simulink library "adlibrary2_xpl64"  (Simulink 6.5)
undefined symbols (not defined in the file or in its folder): Bit, Black, blackbox2, blue, Box, clock_ratio, ddcd732b, gcbh, Inactive, lbif64_xpl_config, Location, Lower, program, VER_STRING_GOES_HERE, white, Width, xbsIndex_r4, xlBlockLoadCallback
libraries: xbsIndex_r4 x49, adlibrary2_xpl64 x1

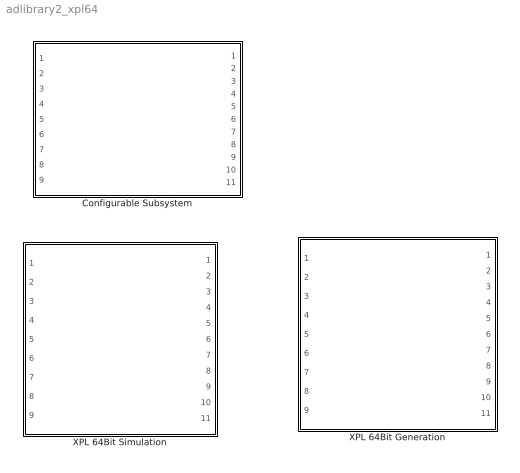
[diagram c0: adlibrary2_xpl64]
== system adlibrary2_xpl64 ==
  Configurable Subsystem : Subsystem  Tag=configX  BlockChoice=XPL 64Bit Simulation  mask{program=program, clock_ratio=clock_ratio}
      mask prompts: program "Local Bus Script Program"; clock_ratio "Clock Ratio"
  XPL 64Bit Generation : Subsystem
  XPL 64Bit Simulation : Subsystem  mask{program=program, clock_ratio=clock_ratio}
      mask prompts: program "Local Bus Script Program"; clock_ratio "Clock Ratio"

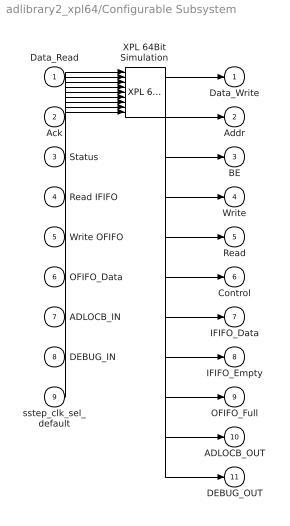
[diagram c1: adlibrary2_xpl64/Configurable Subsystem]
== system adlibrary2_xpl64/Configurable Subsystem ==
  Data_Read : Inport
  Ack : Inport  Port=2
  Status : Inport  Port=3
  Read IFIFO : Inport  Port=4
  Write OFIFO : Inport  Port=5
  OFIFO_Data : Inport  Port=6
  ADLOCB_IN : Inport  Port=7
  DEBUG_IN : Inport  Port=8
  sstep_clk_sel_default : Inport  Port=9
  XPL 64Bit Simulation : adlibrary2_xpl64/XPL 64Bit Simulation  SystemSampleTime=-1  program=program  clock_ratio=clock_ratio
  Data_Write : Outport
  Addr : Outport  Port=2
  BE : Outport  Port=3
  Write : Outport  Port=4
  Read : Outport  Port=5
  Control : Outport  Port=6
  IFIFO_Data : Outport  Port=7
  IFIFO_Empty : Outport  Port=8
  OFIFO_Full : Outport  Port=9
  ADLOCB_OUT : Outport  Port=10
  DEBUG_OUT : Outport  Port=11
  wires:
  Data_Read/1 -> XPL 64Bit Simulation/1
  Ack/1 -> XPL 64Bit Simulation/2
  Status/1 -> XPL 64Bit Simulation/3
  Read IFIFO/1 -> XPL 64Bit Simulation/4
  Write OFIFO/1 -> XPL 64Bit Simulation/5
  OFIFO_Data/1 -> XPL 64Bit Simulation/6
  ADLOCB_IN/1 -> XPL 64Bit Simulation/7
  DEBUG_IN/1 -> XPL 64Bit Simulation/8
  sstep_clk_sel_default/1 -> XPL 64Bit Simulation/9
  XPL 64Bit Simulation/1 -> Data_Write/1
  XPL 64Bit Simulation/2 -> Addr/1
  XPL 64Bit Simulation/3 -> BE/1
  XPL 64Bit Simulation/4 -> Write/1
  XPL 64Bit Simulation/5 -> Read/1
  XPL 64Bit Simulation/6 -> Control/1
  XPL 64Bit Simulation/7 -> IFIFO_Data/1
  XPL 64Bit Simulation/8 -> IFIFO_Empty/1
  XPL 64Bit Simulation/9 -> OFIFO_Full/1
  XPL 64Bit Simulation/10 -> ADLOCB_OUT/1
  XPL 64Bit Simulation/11 -> DEBUG_OUT/1

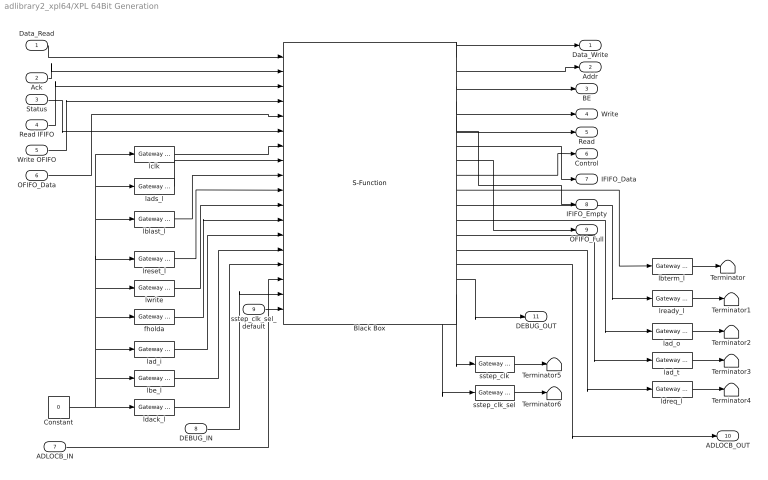
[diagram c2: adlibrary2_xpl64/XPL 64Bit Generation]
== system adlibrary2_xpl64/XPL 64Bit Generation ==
  Data_Read : Inport
  Ack : Inport  Port=2
  Status : Inport  Port=3
  Read IFIFO : Inport  Port=4
  Write OFIFO : Inport  Port=5
  OFIFO_Data : Inport  Port=6
  ADLOCB_IN : Inport  Port=7
  DEBUG_IN : Inport  Port=8
  sstep_clk_sel_default : Inport  Port=9
  Black Box : S-Function  AncestorBlock=xbsIndex_r4/Black Box  LoadFcn=xlBlockLoadCallback(gcbh);  FunctionName=sysgen  Parameters=ptable_  mask(Xilinx Black Box Block){infoedit=Incorporates black box HDL and simulation model into a System Generator design.<P><P>You must supply a Black Box with certain information about the HDL component you would like to bring into System Generator. This information is provided through a Matlab function.<P><P>When "Simulation mode" is set to "Inactive", you will typically want to provide a separate simulation model by using a Simulation 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, init_code=lbif64_xpl_config, sim_method=Inactive, sim_method_sgadvanced=, engine_block=, xl_use_area=on, xl_use_area_sgadvanced=, xl_area=[576,805, 3, 586, 0, 0, 162], block_version=VER_STRING_GOES_HERE, has_advanced_control=0, sggui_pos=20,20,356,367, block_type=blackbox2, sg_icon_stat=240,390,18,18,white,blue,0,ddcd732b, sg_mask_display=fprintf('','COMMENT: begin icon graphics '); patch([0 240 240 0 ],[0 0 390 390 ],[0.77 0.82 0.91]); patch([56 16 72 16 56 119 136 153 221 167 116 79 135 79 116 167 221 153 136 119 56 ],[101 141 197 253 293 293 276 293 293 239 290 253 197 141 104 155 101 101 118 101 101 ],[0.98 0.96 0.92]); plot([0 0 240 240 0 ],[0 390 390 0 0 ]); fprintf('','COMMENT: end icon graphics');  fprintf('','COMMENT: begi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, sg_list_contents=}
      mask prompts: infoedit ""; init_code "Block configuration m-function"; sim_method "Simulation mode"; engine_block "HDL co-simulator to use  (specify helper block by name)"; xl_use_area "Define FPGA area for resource estimation"; xl_area "FPGA area [slices, FFs, BRAMs, LUTs, IOBs, emb. mults, TBUFs]"; block_version ""; has_advanced_control ""; sggui_pos ""; block_type ""; sg_icon_stat ""; sg_mask_display ""; sg_list_contents ""
      mask help: Incorporates black box HDL and simulation model into a System Generator design. You must supply a Black Box with certain information about the HDL component you would like to bring into System Generator. This information is provided through a Matlab function. When "Simulation mode" is set to "Inactive", you will typically want to provide a separate simulation model by using a Simulation Multiplexer. When "Simulation mode" is set to "External co-simulator", you must include a ModelSim block in the design.
      mask init:
      | xlMungeMaskParams;
      | 
      | mdlPath = xlGetMdlDir(bdroot);
      | 
      | refBlk = get_param(gcb,'referenceBlock');
      | if (isempty(refBlk) | strncmp(refBlk,'xbsIndex',8))
      | srcPath = mdlPath;
      | else
      | srcPath = xlPathToReference;
      | if (isempty(srcPath))
      | srcPath = mdlPath;
      | end
      | end
      | 
      | if (sim_method==3)
      | validEngineBlock = 0;
      | try
      | engineBlock = xlBlockNameRelPath(get_param(gcb,'Parent'),engine_block);
      | catch
      | engineBlock = '//';
      | end
      | try 
      | engineWorkDir = get_param(engineBlock,'dir');
      | validEngineBlock = 1;
      | engine_handle = get_param(engineBlock,'Handle');
      | catch
      | end
      | end
      | 
      | % build black box config function
      | block_config = ['sysgen:black_box_config:' init_code];
      | 
      | serialized_declarations = '{''engine_handle''=>''Double'',''sim_method''=>''Int'',''validEngineBlock''=>''Int'',''engineWorkDir''=>''String'',''engine_block''=>''String'',''init_code''=>''String'',''mdlPath''=>''String'',''srcPath''=>''String'',''block_config''=>''String'',}';
      | ptable_ = xlblockprep(get_param(gcb, 'MaskWSVariables'));
  Constant : Constant  Value=0  OutDataType=sfix(16)  ConRadixGroup=Use specified scaling  OutScaling=2^0  SampleTime=inf  FramePeriod=inf
  Terminator{,1..6} (7 alike) : Terminator
  fholda : xbsIndex_r4/Gateway In  arith_type=Boolean  n_bits=8  bin_pt=6  quantization="Round  (unbiased: +/- Inf)"  overflow=Saturate  period=1  dbl_ovrd=off  timing_constraint=None  locs_specified=off  LOCs={}  block_type=gatewayin
  lad_i : xbsIndex_r4/Gateway In  arith_type=Unsigned  n_bits=64  bin_pt=0  quantization="Round  (unbiased: +/- Inf)"  overflow=Saturate  period=1  dbl_ovrd=off  timing_constraint=None  locs_specified=off  LOCs={}  block_type=gatewayin
  lad_o : xbsIndex_r4/Gateway Out  hdl_port=on  timing_constraint=None  locs_specified=off  LOCs={}  block_type=gatewayout
  lad_t : xbsIndex_r4/Gateway Out  hdl_port=on  timing_constraint=None  locs_specified=off  LOCs={}  block_type=gatewayout
  lads_l : xbsIndex_r4/Gateway In  arith_type=Boolean  n_bits=8  bin_pt=6  quantization="Round  (unbiased: +/- Inf)"  overflow=Saturate  period=1  dbl_ovrd=off  timing_constraint=None  locs_specified=off  LOCs={}  block_type=gatewayin
  lbe_l : xbsIndex_r4/Gateway In  arith_type=Unsigned  n_bits=8  bin_pt=0  quantization="Round  (unbiased: +/- Inf)"  overflow=Saturate  period=1  dbl_ovrd=off  timing_constraint=None  locs_specified=off  LOCs={}  block_type=gatewayin
  lblast_l : xbsIndex_r4/Gateway In  arith_type=Boolean  n_bits=8  bin_pt=6  quantization="Round  (unbiased: +/- Inf)"  overflow=Saturate  period=1  dbl_ovrd=off  timing_constraint=None  locs_specified=off  LOCs={}  block_type=gatewayin
  lbterm_l : xbsIndex_r4/Gateway Out  hdl_port=on  timing_constraint=None  locs_specified=off  LOCs={}  block_type=gatewayout
  lclk : xbsIndex_r4/Gateway In  arith_type=Boolean  n_bits=8  bin_pt=6  quantization="Round  (unbiased: +/- Inf)"  overflow=Saturate  period=1  dbl_ovrd=off  timing_constraint=None  locs_specified=off  LOCs={}  block_type=gatewayin
  ldack_l : xbsIndex_r4/Gateway In  arith_type=Unsigned  n_bits=2  bin_pt=0  quantization="Round  (unbiased: +/- Inf)"  overflow=Saturate  period=1  dbl_ovrd=off  timing_constraint=None  locs_specified=off  LOCs={}  block_type=gatewayin
  ldreq_l : xbsIndex_r4/Gateway Out  hdl_port=on  timing_constraint=None  locs_specified=off  LOCs={}  block_type=gatewayout
  lready_l : xbsIndex_r4/Gateway Out  hdl_port=on  timing_constraint=None  locs_specified=off  LOCs={}  block_type=gatewayout
  lreset_l : xbsIndex_r4/Gateway In  arith_type=Boolean  n_bits=8  bin_pt=6  quantization="Round  (unbiased: +/- Inf)"  overflow=Saturate  period=1  dbl_ovrd=off  timing_constraint=None  locs_specified=off  LOCs={}  block_type=gatewayin
  lwrite : xbsIndex_r4/Gateway In  arith_type=Boolean  n_bits=8  bin_pt=6  quantization="Round  (unbiased: +/- Inf)"  overflow=Saturate  period=1  dbl_ovrd=off  timing_constraint=None  locs_specified=off  LOCs={}  block_type=gatewayin
  sstep_clk : xbsIndex_r4/Gateway Out  hdl_port=on  timing_constraint=None  locs_specified=off  LOCs={}  block_type=gatewayout
  sstep_clk_sel : xbsIndex_r4/Gateway Out  hdl_port=on  timing_constraint=None  locs_specified=off  LOCs={}  block_type=gatewayout
  Data_Write : Outport
  Addr : Outport  Port=2
  BE : Outport  Port=3
  Write : Outport  Port=4
  Read : Outport  Port=5
  Control : Outport  Port=6
  IFIFO_Data : Outport  Port=7
  IFIFO_Empty : Outport  Port=8
  OFIFO_Full : Outport  Port=9
  ADLOCB_OUT : Outport  Port=10
  DEBUG_OUT : Outport  Port=11
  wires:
  lbe_l/1 -> Black Box/14
  Data_Read/1 -> Black Box/1
  Ack/1 -> Black Box/2
  Status/1 -> Black Box/6
  Read IFIFO/1 -> Black Box/3
  Write OFIFO/1 -> Black Box/4
  OFIFO_Data/1 -> Black Box/5
  Black Box/1 -> Data_Write/1
  Black Box/2 -> Addr/1
  lclk/1 -> Black Box/7
  lads_l/1 -> Black Box/8
  lblast_l/1 -> Black Box/9
  lreset_l/1 -> Black Box/10
  lwrite/1 -> Black Box/11
  fholda/1 -> Black Box/12
  lad_i/1 -> Black Box/13
  ldack_l/1 -> Black Box/15
  Constant/1 -> ldack_l/1, lclk/1, lads_l/1, lblast_l/1, lreset_l/1, lwrite/1, fholda/1, lad_i/1, lbe_l/1
  lbterm_l/1 -> Terminator/1
  lready_l/1 -> Terminator1/1
  lad_o/1 -> Terminator2/1
  lad_t/1 -> Terminator3/1
  ldreq_l/1 -> Terminator4/1
  Black Box/14 -> ldreq_l/1
  Black Box/3 -> BE/1
  Black Box/4 -> Write/1
  Black Box/5 -> Read/1
  Black Box/6 -> IFIFO_Empty/1
  Black Box/7 -> IFIFO_Data/1
  Black Box/8 -> OFIFO_Full/1
  Black Box/9 -> Control/1
  Black Box/10 -> lbterm_l/1
  Black Box/11 -> lready_l/1
  Black Box/12 -> lad_o/1
  Black Box/13 -> lad_t/1
  Black Box/15 -> ADLOCB_OUT/1
  ADLOCB_IN/1 -> Black Box/16
  sstep_clk/1 -> Terminator5/1
  sstep_clk_sel/1 -> Terminator6/1
  DEBUG_IN/1 -> Black Box/17
  Black Box/17 -> sstep_clk/1
  Black Box/18 -> sstep_clk_sel/1
  Black Box/16 -> DEBUG_OUT/1
  sstep_clk_sel_default/1 -> Black Box/18

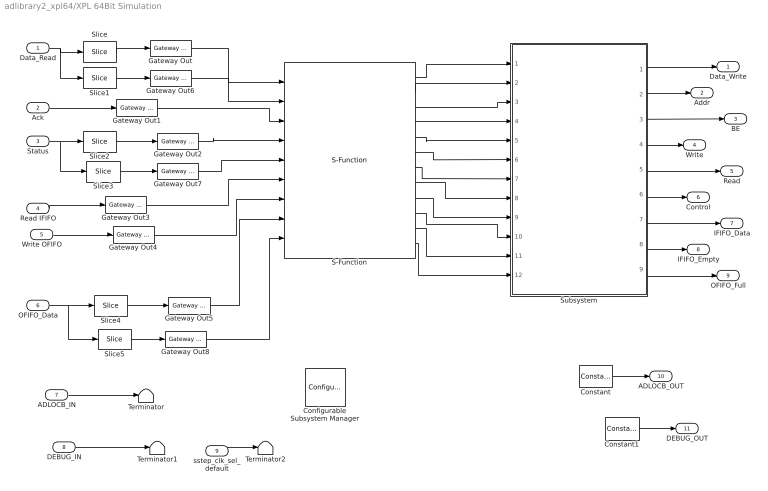
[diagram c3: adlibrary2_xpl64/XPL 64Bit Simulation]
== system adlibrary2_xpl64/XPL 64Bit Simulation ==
  Data_Read : Inport
  Ack : Inport  Port=2
  Status : Inport  Port=3
  Read IFIFO : Inport  Port=4
  Write OFIFO : Inport  Port=5
  OFIFO_Data : Inport  Port=6
  ADLOCB_IN : Inport  Port=7
  DEBUG_IN : Inport  Port=8
  sstep_clk_sel_default : Inport  Port=9
  Configurable Subsystem Manager : xbsIndex_r4/Configurable Subsystem Manager  Tag=xcfgMgr  block_type=configsubsys
  Constant : xbsIndex_r4/Constant  arith_type=Unsigned  const=0  n_bits=66  bin_pt=0  explicit_period=on  period=ad_get_simulink_period  equ=P=C  opselect=C  inp2=PCIN>>17  opr=+  inp1=P  carry=CIN  dbl_ovrd=off  block_type=constant
  Constant1 : xbsIndex_r4/Constant  arith_type=Unsigned  const=0  n_bits=40  bin_pt=0  explicit_period=on  period=ad_get_simulink_period  equ=P=C  opselect=C  inp2=PCIN>>17  opr=+  inp1=P  carry=CIN  dbl_ovrd=off  block_type=constant
  Gateway Out{,1..8} (9 alike) : xbsIndex_r4/Gateway Out  hdl_port=off  timing_constraint=None  locs_specified=off  LOCs={}  block_type=gatewayout
  S-Function : S-Function  FunctionName=lbif_xpl64  Parameters=program,clock_ratio
  Slice : xbsIndex_r4/Slice  nbits=32  boolean_output=off  mode=Lower Bit Location + Width  bit1=0  base1=MSB of Input  bit0=0  base0=LSB of Input  dbl_ovrd=off  block_type=slice
  Slice1 : xbsIndex_r4/Slice  nbits=32  boolean_output=off  mode=Lower Bit Location + Width  bit1=0  base1=MSB of Input  bit0=32  base0=LSB of Input  dbl_ovrd=off  block_type=slice
  Slice2 : xbsIndex_r4/Slice  nbits=32  boolean_output=off  mode=Lower Bit Location + Width  bit1=0  base1=MSB of Input  bit0=0  base0=LSB of Input  dbl_ovrd=off  block_type=slice
  Slice3 : xbsIndex_r4/Slice  nbits=32  boolean_output=off  mode=Lower Bit Location + Width  bit1=0  base1=MSB of Input  bit0=32  base0=LSB of Input  dbl_ovrd=off  block_type=slice
  Slice4 : xbsIndex_r4/Slice  nbits=32  boolean_output=off  mode=Lower Bit Location + Width  bit1=0  base1=MSB of Input  bit0=0  base0=LSB of Input  dbl_ovrd=off  block_type=slice
  Slice5 : xbsIndex_r4/Slice  nbits=32  boolean_output=off  mode=Lower Bit Location + Width  bit1=0  base1=MSB of Input  bit0=32  base0=LSB of Input  dbl_ovrd=off  block_type=slice
  Subsystem : Subsystem
  Terminator : Terminator
  Terminator1 : Terminator
  Terminator2 : Terminator
  Data_Write : Outport
  Addr : Outport  Port=2
  BE : Outport  Port=3
  Write : Outport  Port=4
  Read : Outport  Port=5
  Control : Outport  Port=6
  IFIFO_Data : Outport  Port=7
  IFIFO_Empty : Outport  Port=8
  OFIFO_Full : Outport  Port=9
  ADLOCB_OUT : Outport  Port=10
  DEBUG_OUT : Outport  Port=11
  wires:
  Data_Read/1 -> Slice/1, Slice1/1
  Ack/1 -> Gateway Out1/1
  Status/1 -> Slice2/1, Slice3/1
  Read IFIFO/1 -> Gateway Out3/1
  Write OFIFO/1 -> Gateway Out4/1
  OFIFO_Data/1 -> Slice4/1, Slice5/1
  Slice/1 -> Gateway Out/1
  Slice1/1 -> Gateway Out6/1
  Gateway Out/1 -> S-Function/1
  Gateway Out6/1 -> S-Function/2
  Gateway Out1/1 -> S-Function/3
  Slice2/1 -> Gateway Out2/1
  Slice3/1 -> Gateway Out7/1
  Gateway Out2/1 -> S-Function/4
  Gateway Out7/1 -> S-Function/5
  Gateway Out3/1 -> S-Function/6
  Gateway Out4/1 -> S-Function/7
  Slice4/1 -> Gateway Out5/1
  Slice5/1 -> Gateway Out8/1
  Gateway Out5/1 -> S-Function/8
  Gateway Out8/1 -> S-Function/9
  S-Function/1 -> Subsystem/1(data_write0)
  S-Function/2 -> Subsystem/2(data_write1)
  S-Function/3 -> Subsystem/3(addr)
  S-Function/4 -> Subsystem/4(be)
  S-Function/5 -> Subsystem/5(write)
  S-Function/6 -> Subsystem/6(read)
  S-Function/7 -> Subsystem/7(control0)
  S-Function/8 -> Subsystem/8(control1)
  S-Function/9 -> Subsystem/9(ififo_data0)
  S-Function/12 -> Subsystem/12(ofifo_full)
  S-Function/11 -> Subsystem/11(ififo_empty)
  S-Function/10 -> Subsystem/10(ififo_data1)
  Subsystem/9(Out9) -> OFIFO_Full/1
  Subsystem/8(Out8) -> IFIFO_Empty/1
  Subsystem/7(Out7) -> IFIFO_Data/1
  Subsystem/6(Out6) -> Control/1
  Subsystem/5(Out5) -> Read/1
  Subsystem/4(Out4) -> Write/1
  Subsystem/3(Out3) -> BE/1
  Subsystem/2(Out2) -> Addr/1
  Subsystem/1(Out1) -> Data_Write/1
  ADLOCB_IN/1 -> Terminator/1
  Constant/1 -> ADLOCB_OUT/1
  DEBUG_IN/1 -> Terminator1/1
  Constant1/1 -> DEBUG_OUT/1
  sstep_clk_sel_default/1 -> Terminator2/1

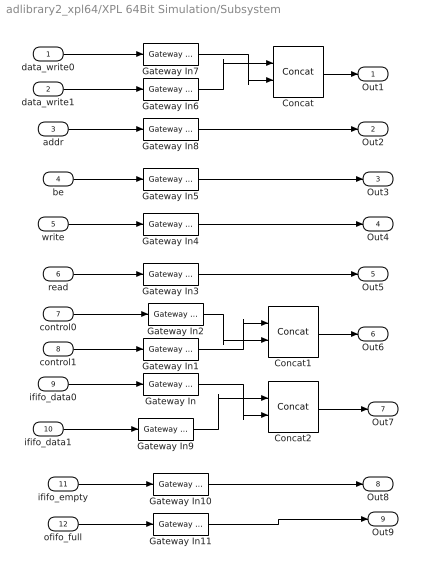
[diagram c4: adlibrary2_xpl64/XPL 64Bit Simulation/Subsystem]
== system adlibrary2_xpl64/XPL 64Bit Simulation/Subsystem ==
  data_write0 : Inport
  data_write1 : Inport  Port=2
  addr : Inport  Port=3
  be : Inport  Port=4
  write : Inport  Port=5
  read : Inport  Port=6
  control0 : Inport  Port=7
  control1 : Inport  Port=8
  ififo_data0 : Inport  Port=9
  ififo_data1 : Inport  Port=10
  ififo_empty : Inport  Port=11
  ofifo_full : Inport  Port=12
  Concat : xbsIndex_r4/Concat  num_inputs=2  dbl_ovrd=off  block_type=concat
  Concat1 : xbsIndex_r4/Concat  num_inputs=2  dbl_ovrd=off  block_type=concat
  Concat2 : xbsIndex_r4/Concat  num_inputs=2  dbl_ovrd=off  block_type=concat
  Gateway In{,1..2,6..7,9} (6 alike) : xbsIndex_r4/Gateway In  arith_type=Unsigned  n_bits=32  bin_pt=0  quantization="Round  (unbiased: +/- Inf)"  overflow=Saturate  period=ad_get_simulink_period  dbl_ovrd=off  timing_constraint=None  locs_specified=off  LOCs={}  block_type=gatewayin
  Gateway In10 : xbsIndex_r4/Gateway In  arith_type=Boolean  n_bits=8  bin_pt=6  quantization="Round  (unbiased: +/- Inf)"  overflow=Saturate  period=ad_get_simulink_period  dbl_ovrd=off  timing_constraint=None  locs_specified=off  LOCs={}  block_type=gatewayin
  Gateway In11 : xbsIndex_r4/Gateway In  arith_type=Boolean  n_bits=8  bin_pt=6  quantization="Round  (unbiased: +/- Inf)"  overflow=Saturate  period=ad_get_simulink_period  dbl_ovrd=off  timing_constraint=None  locs_specified=off  LOCs={}  block_type=gatewayin
  Gateway In3 : xbsIndex_r4/Gateway In  arith_type=Boolean  n_bits=32  bin_pt=0  quantization="Round  (unbiased: +/- Inf)"  overflow=Saturate  period=ad_get_simulink_period  dbl_ovrd=off  timing_constraint=None  locs_specified=off  LOCs={}  block_type=gatewayin
  Gateway In4 : xbsIndex_r4/Gateway In  arith_type=Boolean  n_bits=8  bin_pt=6  quantization="Round  (unbiased: +/- Inf)"  overflow=Saturate  period=ad_get_simulink_period  dbl_ovrd=off  timing_constraint=None  locs_specified=off  LOCs={}  block_type=gatewayin
  Gateway In5 : xbsIndex_r4/Gateway In  arith_type=Unsigned  n_bits=8  bin_pt=0  quantization="Round  (unbiased: +/- Inf)"  overflow=Saturate  period=ad_get_simulink_period  dbl_ovrd=off  timing_constraint=None  locs_specified=off  LOCs={}  block_type=gatewayin
  Gateway In8 : xbsIndex_r4/Gateway In  arith_type=Unsigned  n_bits=16  bin_pt=0  quantization="Round  (unbiased: +/- Inf)"  overflow=Saturate  period=ad_get_simulink_period  dbl_ovrd=off  timing_constraint=None  locs_specified=off  LOCs={}  block_type=gatewayin
  Out1 : Outport
  Out2 : Outport  Port=2
  Out3 : Outport  Port=3
  Out4 : Outport  Port=4
  Out5 : Outport  Port=5
  Out6 : Outport  Port=6
  Out7 : Outport  Port=7
  Out8 : Outport  Port=8
  Out9 : Outport  Port=9
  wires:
  data_write0/1 -> Gateway In7/1
  data_write1/1 -> Gateway In6/1
  be/1 -> Gateway In5/1
  write/1 -> Gateway In4/1
  read/1 -> Gateway In3/1
  control0/1 -> Gateway In2/1
  control1/1 -> Gateway In1/1
  ififo_data0/1 -> Gateway In/1
  addr/1 -> Gateway In8/1
  Gateway In6/1 -> Concat/1
  Gateway In7/1 -> Concat/2
  Concat/1 -> Out1/1
  Gateway In8/1 -> Out2/1
  Gateway In5/1 -> Out3/1
  Gateway In4/1 -> Out4/1
  Gateway In3/1 -> Out5/1
  Gateway In2/1 -> Concat1/2
  Gateway In1/1 -> Concat1/1
  Concat1/1 -> Out6/1
  ififo_data1/1 -> Gateway In9/1
  ififo_empty/1 -> Gateway In10/1
  ofifo_full/1 -> Gateway In11/1
  Gateway In9/1 -> Concat2/1
  Gateway In/1 -> Concat2/2
  Concat2/1 -> Out7/1
  Gateway In10/1 -> Out8/1
  Gateway In11/1 -> Out9/1
